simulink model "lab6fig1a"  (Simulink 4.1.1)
settings: Solver=ode45  SolverMode=SingleTasking  StartTime=0.0  StopTime=10.0  MaxStep=2e-3  RelTol=1e-6  AbsTol=1e-6

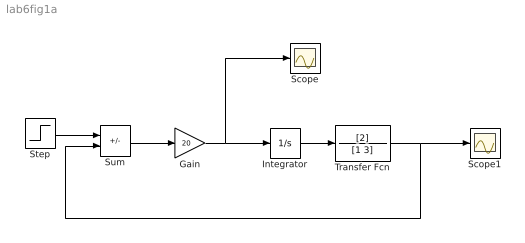
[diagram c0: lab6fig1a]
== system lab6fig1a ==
  Gain : Gain  Gain=20  Multiplication=Element-wise(K.*u)  SaturateOnIntegerOverflow=on
  Integrator : Integrator  ExternalReset=none  InitialConditionSource=internal  InitialCondition=0  LimitOutput=off  UpperSaturationLimit=inf  LowerSaturationLimit=-inf  ShowSaturationPort=off  ShowStatePort=off  AbsoluteTolerance=auto
  Scope : Scope
  Scope1 : Scope
  Step : Step  Time=0  Before=0  After=1  SampleTime=-1
  Sum : Sum  Inputs=+-  SaturateOnIntegerOverflow=on
  Transfer Fcn : TransferFcn  Numerator=[2]  Denominator=[1 3]  AbsoluteTolerance=auto  Realization=auto
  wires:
  Step/1 -> Sum/1
  Sum/1 -> Gain/1
  Integrator/1 -> Transfer Fcn/1
  Gain/1 -> Integrator/1, Scope/1
  Transfer Fcn/1 -> Scope1/1, Sum/2
